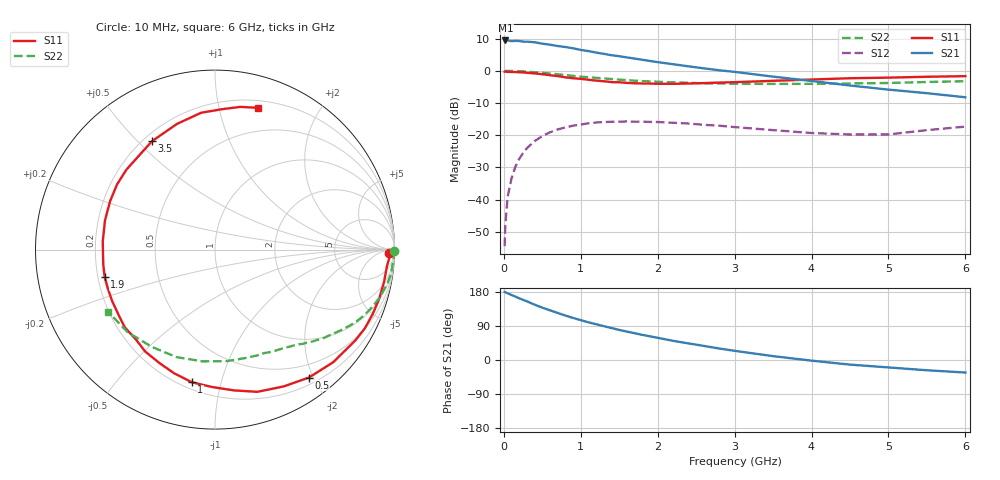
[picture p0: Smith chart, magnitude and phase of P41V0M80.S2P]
! SIEMENS Small Signal Semiconductors
! BFP182
! Si NPN RF Bipolar Junction Transistor in SOT143
! VCE = 1 V  IC = 0.8 mA
! Common Emitter S-Parameters:  March  1996
# GHz  S  MA  R  50
!  f  S11  S21  S12  S22
! GHz  MAG  ANG  MAG  ANG  MAG  ANG  MAG  ANG
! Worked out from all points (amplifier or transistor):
!   36 points, 10 MHz to 6 GHz, reference 50 ohm
!   highest |S21| = 9.4 dB at 20 MHz (marker M1)
!   |S21| within 3 dB of that: start of sweep to 1.018 GHz
!   unconditionally stable (mu >= 1): 2.656 GHz to end of sweep
!   at 250 MHz: K = 0.09, MSG = 17.3 dB, |S12| = -25.5 dB
!   at 1.4 GHz: K = 0.54, MSG = 10.3 dB, |S12| = -15.8 dB
!   at 6 GHz: K = 1.26, MAG = 1.5 dB, |S12| = -17.3 dB
!   S11 on the Smith chart (normalised r, x): 10 MHz: 46, -28; 500 MHz: 0.30, -1.94; 1 GHz: 0.24, -0.81; 1.9 GHz: 0.23, -0.11; 3.5 GHz: 0.23, +0.55; 6 GHz: 0.26, +1.31
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0.01  0.9686 -1.1  2.891 179.6  0.0019 92.2  0.9985 -0.4
0.02  0.9741 -2.3  2.954 178.9  0.0042 91.2  0.9913 -0.9
0.05  0.9622 -5.6  2.953 175.8  0.0112 89.1  0.9971 -2.2
0.1  0.9591 -10.8  2.882 171.6  0.0214 83.1  0.9934 -4.4
0.15  0.955 -16.7  2.912 167.2  0.0324 79.2  0.9909 -6.6
0.25  0.9433 -27.6  2.836 158.6  0.0529 72.6  0.9795 -11.0
0.3  0.9315 -32.9  2.83 154.9  0.0629 69.0  0.9704 -12.9
0.4  0.9097 -43.6  2.769 146.0  0.0809 62.3  0.9514 -16.9
0.5  0.8843 -53.7  2.633 138.2  0.0971 56.2  0.929 -20.6
0.6  0.8531 -63.3  2.539 131.1  0.1111 50.3  0.9067 -24.0
0.8  0.792 -82.2  2.338 117.3  0.1323 39.8  0.8576 -29.9
1  0.7502 -99.9  2.107 105.2  0.1467 30.4  0.8113 -35.1
1.1  0.7253 -108.4  2.019 99.4  0.1531 26.5  0.7933 -37.3
1.5  0.6637 -139.1  1.684 79.4  0.1623 12.6  0.7285 -45.3
1.9  0.6333 -166.2  1.419 62.5  0.1609 2.6  0.6831 -52.3
2.2  0.627 175.8  1.264 50.6  0.1559 -3.2  0.6612 -57.4
2.8  0.6556 146.3  1.018 30.3  0.1406 -11.3  0.6344 -68.4
3.5  0.6985 120.2  0.811 10.2  0.12 -14.2  0.6249 -83.8
4.5  0.7663 95.8  0.591 -12.2  0.1027 -6.3  0.6363 -109.7
5  0.7826 87.4  0.51 -19.6  0.1029 3.6  0.6462 -123.0
5.5  0.8074 80.0  0.449 -27.1  0.12 7.7  0.6699 -136.7
6  0.8253 73.2  0.388 -33.1  0.136 8.1  0.6887 -149.7
